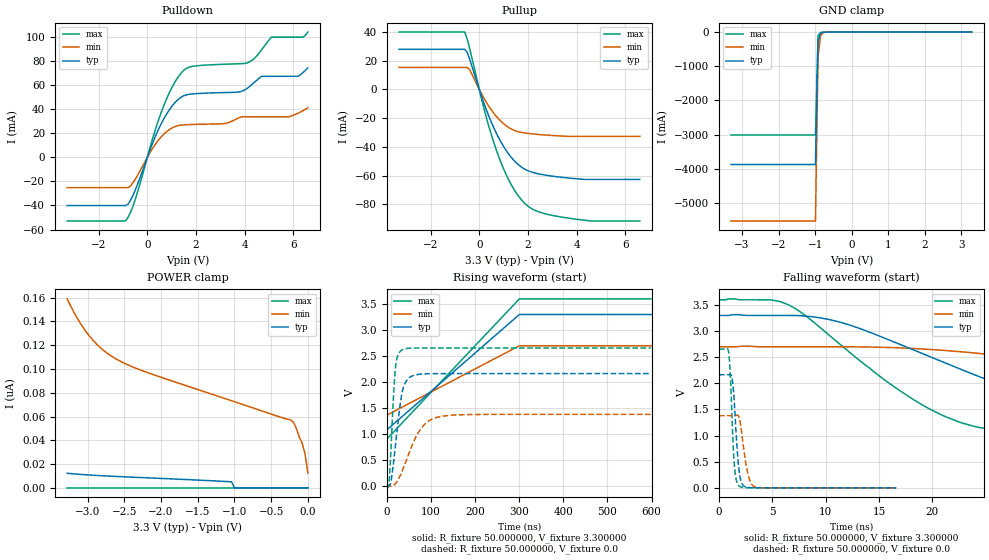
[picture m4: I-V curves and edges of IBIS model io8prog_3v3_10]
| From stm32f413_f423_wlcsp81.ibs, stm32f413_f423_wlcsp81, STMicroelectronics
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|   Model io8prog_3v3_10
[Model]  io8prog_3v3_10
Model_type I/O
Polarity   Non-Inverting
Enable   Active-Low
Vinl =   0.990000V
Vinh =   2.310000V
Vmeas =  1.650000V
Cref =   100.000000pF
Rref =   1.000000k
Vref =   3.300000V
C_comp   2.665600pF   2.506300pF   2.859000pF
[Temperature Range]   25.000000   0.125000k   -40.000000
[Pullup Reference]   3.300000V   2.700000V   3.600000V
[Pulldown Reference]   0.0V   0.0V   0.0V
[POWER Clamp Reference]   3.300000V   2.700000V   3.600000V
[GND Clamp Reference]   0.0V   0.0V   0.0V
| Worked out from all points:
|   slope of the pulldown table from 0 to 0.495 V, typ, clamps not added: 20 ohm
|   slope of the pullup table from 0 to 0.495 V, typ, clamps not added: 21.7 ohm
|   GND clamp passes 1 mA (typ) near -0.57 V on its own axis
|   rising waveform, R_fixture 50.000000, V_fixture 3.300000: 20-80 % time 180ns typ, 180ns min, 180ns max; typ from 1.09 V to 3.3 V
|   rising waveform, R_fixture 50.000000, V_fixture 0.0: 20-80 % time 18.3ns typ, 43.3ns min, 9.75ns max; typ from 0 V to 2.17 V
|   falling waveform, R_fixture 50.000000, V_fixture 3.300000: 20-80 % time 17.4ns typ, 34.6ns min, 10.8ns max; typ from 3.3 V to 1.09 V
|   falling waveform, R_fixture 50.000000, V_fixture 0.0: 20-80 % time 422ps typ, 611ps min, 335ps max; typ from 2.17 V to 0 V
[Pulldown]
|Voltage   I(typ)   I(min)   I(max)
-3.3V     -40.11mA   -25.24mA   -52.93mA
-900mV    -40.11mA   -25.24mA   -52.93mA
-500mV    -27.39mA   -18.31mA   -35.21mA
600mV     29.01mA    17.61mA    38.88mA
1.1V      44.56mA    25.16mA    61.26mA
1.5V      51.11mA    26.89mA    72.21mA
3.1V      53.67mA    27.79mA    77.15mA
4.1V      57.11mA    33.57mA    78.25mA
4.7V      67.22mA    33.57mA    89.26mA
5.1V      67.22mA    33.57mA    99.69mA
6.2V      67.22mA    36.63mA    99.69mA
6.6V      74.18mA    41.08mA    104mA
[Pullup]
|Voltage   I(typ)   I(min)   I(max)
-3.3V     27.94mA    15.3mA     39.98mA
-600mV    27.94mA    15.3mA     39.98mA
-500mV    25.89mA    15.3mA     35.29mA
-400mV    21.3mA     13.82mA    28.75mA
300mV     -14.62mA   -9.248mA   -20.15mA
800mV     -33.8mA    -20.67mA   -46.89mA
1.1V      -42.41mA   -25.28mA   -59.19mA
1.4V      -49.01mA   -28.29mA   -68.91mA
2V        -56.64mA   -30.64mA   -81.32mA
2.6V      -59.37mA   -31.63mA   -86.14mA
3.9V      -62.11mA   -32.7mA    -90.25mA
6.6V      -62.7mA    -32.7mA    -91.7mA
[GND_clamp]
|Voltage   I(typ)   I(min)   I(max)
-3.3V     -3.872A    -5.523A    -3.009A
-990mV    -3.872A    -5.523A    -3.009A
-920mV    -262.2mA   -719.6mA   -104.3mA
-850mV    -25.19mA   -100.9mA   -13.07mA
-780mV    -6.959mA   -18mA      -7.19mA
3.28V     0A         5.62nA     0A
[POWER_clamp]
|Voltage   I(typ)   I(min)   I(max)
-3.28V    12.27nA    159nA      0A
-3.12V    11.41nA    140.5nA    0A
-2.96V    10.73nA    126.5nA    0A
-2.76V    10.05nA    114.5nA    0A
-2.56V    9.455nA    106.7nA    0A
-1.04V    5.085nA    73.31nA    0A
-1V       0A         72.48nA    0A
-240mV    0A         57.24nA    0A
-200mV    0A         55.42nA    0A
-80mV     0A         37.96nA    0A
-40mV     0A         28.96nA    0A
0V        0A         12.44nA    0A
[Ramp]
| variable   typ   min   max
dV/dt_r  1.29876/18.26930n   0.82878/43.28389n   1.59366/9.73351n
dV/dt_f  1.32768/17.42868n   0.79902/35.60785n   1.61434/10.81937n
R_load = 50.000000
[Rising Waveform]
R_fixture= 50.000000
V_fixture= 3.300000
V_fixture_min= 2.700000
V_fixture_max= 3.600000
|time   V(typ)   V(min)   V(max)
0s        1.087V     1.368V     909.4mV
300.3ns   3.3V       2.7V       3.6V
600.6ns   3.3V       2.7V       3.6V
29.73us   3.3V       2.7V       3.6V
[Rising Waveform]
R_fixture= 50.000000
V_fixture= 0.0
V_fixture_min= 0.0
V_fixture_max= 0.0
|time   V(typ)   V(min)   V(max)
0s        3.921nV    214.3nV    2.7nV
4.805ns   3.881mV    -154.2uV   84.77mV
10.81ns   183mV      2.957mV    1.041V
19.22ns   792.3mV    54.55mV    2.283V
25.23ns   1.25V      125mV      2.526V
34.83ns   1.822V     301.8mV    2.623V
49.25ns   2.077V     619.8mV    2.651V
70.87ns   2.148V     1.03V      2.656V
111.7ns   2.164V     1.321V     2.656V
598.2ns   2.165V     1.381V     2.656V
[Falling Waveform]
R_fixture= 50.000000
V_fixture= 3.300000
V_fixture_min= 2.700000
V_fixture_max= 3.600000
|time   V(typ)   V(min)   V(max)
0s        3.3V       2.7V       3.6V
6.607ns   3.3V       2.7V       3.495V
11.41ns   3.169V     2.7V       2.737V
19.82ns   2.508V     2.649V     1.501V
24.02ns   2.159V     2.581V     1.173V
27.93ns   1.853V     2.494V     1.062V
33.63ns   1.502V     2.35V      995.1mV
40.54ns   1.299V     2.162V     956.9mV
70.27ns   1.123V     1.579V     915.2mV
149.5ns   1.087V     1.368V     909.4mV
[Falling Waveform]
R_fixture= 50.000000
V_fixture= 0.0
V_fixture_min= 0.0
V_fixture_max= 0.0
|time   V(typ)   V(min)   V(max)
0s        2.165V     1.381V     2.656V
900.9ps   2.165V     1.381V     2.608V
1.101ns   2.171V     1.381V     2.048V
1.235ns   2.096V     1.381V     1.306V
1.468ns   1.553V     1.383V     387.2mV
1.735ns   670.6mV    1.391V     84.79mV
1.969ns   222.6mV    1.281V     24.26mV
2.669ns   9.043mV    317.4mV    2.225mV
3.337ns   1.427mV    23.84mV    1.283mV
16.62ns   3.921nV    214.3nV    2.7nV
